FUNCTION_BLOCK "Main"
VERSION : 0.1
   VAR_INPUT
      in1 : Bool;
   END_VAR

   VAR_OUTPUT
      out1 : Bool;
   END_VAR


BEGIN
NETWORK
TITLE =
      CLR;
      X #in1;
      XN #in1;
      = #out1;
      CALL "__CPROVER_assert"
      (  condition := #out1
      );

END_FUNCTION_BLOCK

